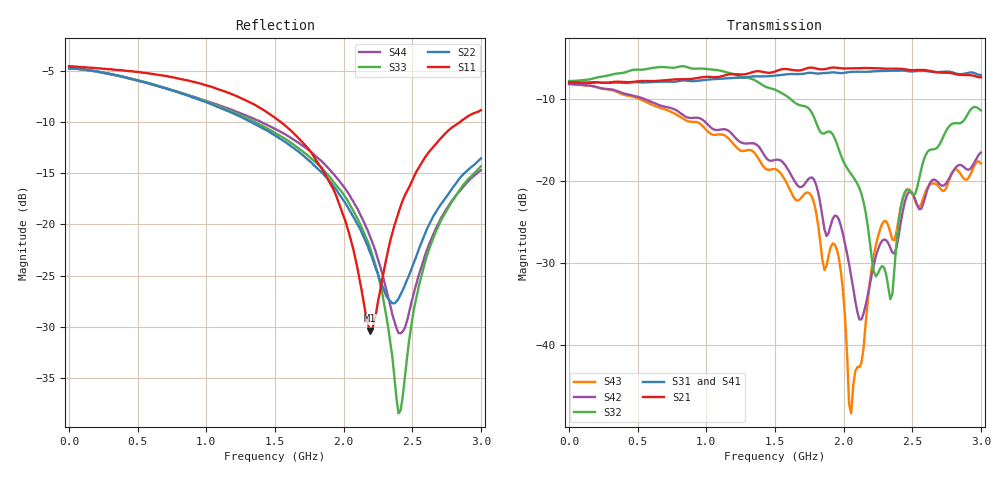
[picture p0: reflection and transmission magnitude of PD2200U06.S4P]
!Agilent Technologies,E5071C,MY46103565,A.11.31
!Date: Fri Mar 24 03:18:40 2017
!Data & Calibration Information:
!Freq	S11:SOLT4(ON)	S12:SOLT4(ON)	S13:SOLT4(ON)	S14:SOLT4(ON)
!	S21:SOLT4(ON)	S22:SOLT4(ON)	S23:SOLT4(ON)	S24:SOLT4(ON)
!	S31:SOLT4(ON)	S32:SOLT4(ON)	S33:SOLT4(ON)	S34:SOLT4(ON)
!	S41:SOLT4(ON)	S42:SOLT4(ON)	S43:SOLT4(ON)	S44:SOLT4(ON)
!PortZ  Port1:50+j0  Port2:50+j0  Port3:50+j0  Port4:50+j0
!Above PortZ is port z conversion or system Z0 setting when saving the data.
!When reading, reference impedance value at option line is always used.
# Hz S dB R 50
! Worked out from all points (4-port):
!   201 points, 1 MHz to 3 GHz, reference 50 ohm
!   strongest paths, dB at 1 MHz, 750.8 MHz, 1.5 GHz, 2.25 GHz, 3 GHz:
!     S21: -8.0, -7.7, -6.7, -6.3, -7.4
!     S31: -8.0, -7.9, -7.2, -6.6, -7.1
!     S41: -8.0, -7.8, -7.1, -6.7, -7.4
!     S32: -7.9, -6.2, -8.9, -31.3, -11.4
!     S42: -8.2, -11.2, -17.4, -28.4, -16.6
!     S43: -8.2, -11.7, -18.6, -26.8, -17.9
!   lowest |S11| = -30.3 dB at 2.19 GHz (marker M1), VSWR 1.06, Z = 47.4 + j1.34 ohm
!   |S11| at or under -10 dB: 1.541 GHz to 2.849 GHz (1.309 GHz wide, 59.6 % of centre)
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1000000  -4.58 179.8  -8.00 -0.1  -8.01 -0.2  -8.01 -0.1
         -8.01 -0.2  -4.77 179.8  -7.85 -0.0  -8.21 -0.2
         -8.02 -0.1  -7.85 -0.0  -4.78 179.7  -8.23 -0.2
         -8.02 -0.2  -8.22 -0.2  -8.23 -0.1  -4.78 179.7
7.95735e8  -5.78 75.2  -7.52 -96.1  -7.86 -98.1  -7.75 -98.2
           -7.65 -95.8  -7.12 15.3  -6.18 -83.4  -11.57 -138.5
           -7.87 -97.6  -6.14 -82.3  -7.09 16.8  -12.01 -127.5
           -7.79 -98.0  -11.55 -139.0  -12.06 -128.7  -7.10 17.3
1.755415e9  -12.81 -66.2  -6.69 139.1  -7.20 136.6  -7.22 139.3
            -6.22 137.7  -13.84 -171.2  -11.23 144.5  -19.58 73.2
            -6.85 135.9  -11.35 144.7  -13.47 -173.4  -21.70 95.9
            -6.73 137.3  -19.61 72.9  -21.55 94.9  -12.85 -170.9
2.055315e9  -21.64 -125.7  -6.23 94.9  -6.72 94.7  -6.71 95.6
            -6.32 94.5  -18.87 136.5  -19.17 113.4  -32.08 -22.3
            -6.74 94.2  -19.17 112.4  -18.30 128.2  -49.98 -122.1
            -6.80 95.6  -31.56 -21.6  -48.25 -124.8  -17.43 135.1
2.19027e9  -30.34 152.3  -6.27 75.1  -6.69 74.5  -6.72 76.0
           -6.28 74.8  -22.66 122.6  -27.21 96.6  -32.72 -91.4
           -6.71 74.8  -27.31 94.8  -22.16 104.6  -32.51 -134.7
           -6.70 75.8  -32.65 -88.2  -32.40 -136.5  -21.09 115.8
2.4002e9  -18.84 36.2  -6.52 43.4  -6.75 42.9  -6.85 45.4
          -6.36 43.7  -27.24 154.0  -24.71 -132.4  -26.53 177.1
          -6.60 43.6  -25.15 -132.4  -38.40 132.7  -24.68 -178.2
          -6.68 45.2  -26.75 173.3  -24.66 -179.2  -30.58 136.8
3e9  -8.86 -71.0  -6.61 -40.6  -6.35 -42.5  -6.49 -39.8
     -7.40 -44.2  -13.57 114.0  -11.48 144.7  -16.58 50.5
     -7.13 -46.2  -11.43 144.5  -14.33 129.8  -17.84 75.5
     -7.40 -41.5  -16.56 52.0  -17.85 75.9  -14.72 127.8
